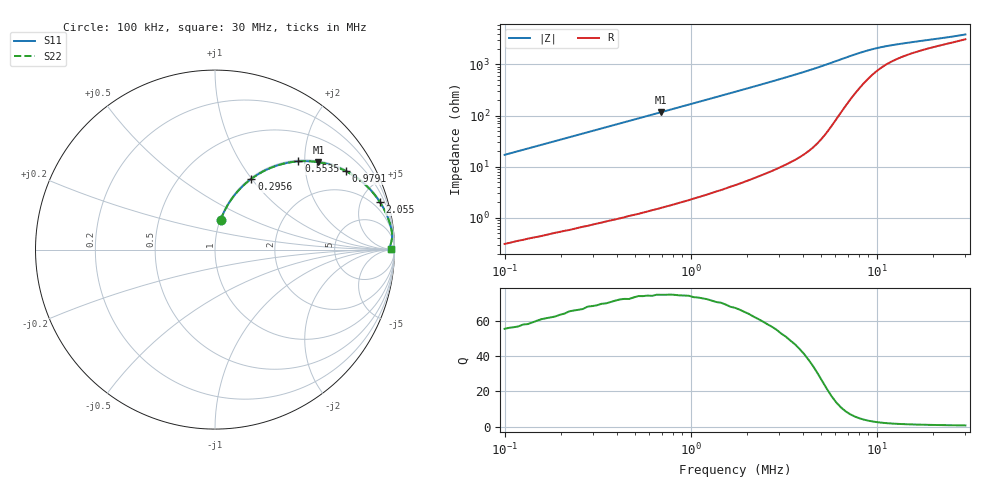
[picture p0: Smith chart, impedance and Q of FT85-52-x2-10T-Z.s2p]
! ListType=Log
!!FT85-52 x2 10T Z
# MHZ S RI R 50
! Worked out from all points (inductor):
!   101 points, 100 kHz to 30 MHz, reference 50 ohm
!   read as one part in series: L = 27.1 uH near 100 kHz
!   highest Q = 74.5 at 695.4 kHz (marker M1), where L = 26.7 uH
!   S11 on the Smith chart (normalised r, x): 100 kHz: 1.01, +0.34; 295.6 kHz: 1.02, +1.00; 553.5 kHz: 1.03, +1.86; 979.1 kHz: 1.05, +3.29; 2.055 MHz: 1.12, +6.96; 30 MHz: 92, +15
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0.1  0.0313 0.1648  0.969 -0.1649  0.9691 -0.1648  0.0312 0.1646
0.1330014  0.0522 0.2136  0.9481 -0.2138  0.9482 -0.2136  0.0521 0.2134
0.1670863  0.0783 0.2602  0.922 -0.2604  0.9222 -0.2602  0.0781 0.26
0.2099064  0.1162 0.3125  0.884 -0.3127  0.8842 -0.3124  0.116 0.3122
0.2637003  0.1697 0.3676  0.8306 -0.3679  0.8309 -0.3677  0.1694 0.3673
0.295565  0.2032 0.3947  0.7971 -0.3951  0.7974 -0.3949  0.2028 0.3945
0.350725  0.2625 0.4325  0.7379 -0.4329  0.7382 -0.4327  0.2621 0.4323
0.4161791  0.332 0.4637  0.6683 -0.4642  0.6687 -0.464  0.3315 0.4635
0.5535239  0.4649 0.4916  0.5353 -0.4923  0.5358 -0.4922  0.4644 0.4916
0.6953784  0.5762 0.487  0.4239 -0.4878  0.4244 -0.4878  0.5757 0.4872
0.8251537  0.6555 0.4681  0.3446 -0.4688  0.345 -0.469  0.6551 0.4682
0.9791484  0.7271 0.4382  0.2729 -0.439  0.2733 -0.4392  0.7267 0.4384
1.302281  0.8236 0.3736  0.1763 -0.3745  0.1766 -0.3747  0.8233 0.3738
1.833715  0.9015 0.2896  0.0983 -0.2907  0.0985 -0.2909  0.9013 0.2899
2.055296  0.9197 0.2631  0.0801 -0.2641  0.0802 -0.2643  0.9196 0.2633
2.89402  0.9574 0.1918  0.0424 -0.1931  0.0425 -0.1933  0.9573 0.192
4.567423  0.9819 0.1177  0.0179 -0.1196  0.018 -0.1198  0.9819 0.1178
6.431296  0.9867 0.0748  0.0131 -0.0774  0.0131 -0.0775  0.9867 0.0749
8.553711  0.9837 0.0493  0.016 -0.0527  0.016 -0.0527  0.9837 0.0494
10.15005  0.981 0.0386  0.0187 -0.0426  0.0187 -0.0426  0.981 0.0386
12.04431  0.9788 0.0307  0.0209 -0.0355  0.0209 -0.0355  0.9789 0.0307
30  0.979 0.0033  0.0205 -0.0149  0.0205 -0.0149  0.9791 0.00329
